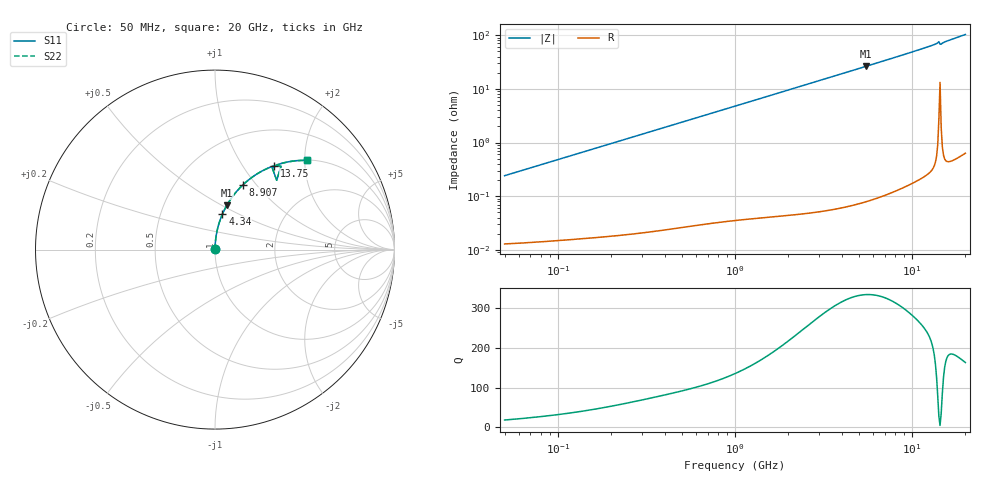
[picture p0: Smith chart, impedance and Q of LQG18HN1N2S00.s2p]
!Murata Part Number: LQG18HN1N2S00
!These Parameters are Measured in Series Mode Connection
!  o--[Z]--o
!Port1  Port2
!  o-------o
!Freq. Start=50[MHz] Stop=20[GHz], 401[Steps]
# Hz S RI R 50
!Freq.(Hz) S11(Real) S11(Imag) S21(Real) S21(Imag) S12(Real) S12(Imag) S22(Real) S22(Imag)
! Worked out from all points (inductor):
!   401 points, 50 MHz to 20 GHz, reference 50 ohm
!   read as one part in series: L = 767 pH near 51.52 MHz
!   highest Q = 332 at 5.516 GHz (marker M1), where L = 760 pH
!   S11 on the Smith chart (normalised r, x): 50 MHz: 1.00, +0.00; 4.34 GHz: 1.00, +0.41; 8.907 GHz: 1.00, +0.86; 13.75 GHz: 1.01, +1.39; 20 GHz: 1.01, +2.06
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5e7  0.000135 0.00241  0.9999 -0.00241  0.9999 -0.00241  0.000135 0.00241
1.364002e8  0.000204 0.00654  0.9998 -0.00654  0.9998 -0.00654  0.000204 0.00654
3.721004e8  0.000543 0.0178  0.9995 -0.0178  0.9995 -0.0178  0.000543 0.0178
1e9  0.00261 0.0474  0.9974 -0.0474  0.9974 -0.0474  0.00261 0.0474
1.714689e9  0.007 0.0809  0.993 -0.0809  0.993 -0.0809  0.007 0.0809
2.728004e9  0.017 0.1274  0.983 -0.1274  0.983 -0.1274  0.017 0.1274
4.34015e9  0.0416 0.198  0.9584 -0.198  0.9584 -0.198  0.0416 0.198
5.515528e9  0.0655 0.2459  0.9345 -0.2459  0.9345 -0.2459  0.0655 0.2459
7.442007e9  0.114 0.3163  0.886 -0.3163  0.886 -0.3163  0.114 0.3163
8.907419e9  0.157 0.3621  0.843 -0.3621  0.843 -0.3621  0.157 0.3621
1.019291e10  0.1979 0.3966  0.8021 -0.3966  0.8021 -0.3966  0.1979 0.3966
1.166392e10  0.2473 0.4295  0.7527 -0.4295  0.7527 -0.4295  0.2473 0.4295
1.314879e10  0.301 0.4562  0.699 -0.4562  0.699 -0.4562  0.301 0.4562
1.375312e10  0.3281 0.4655  0.6719 -0.4655  0.6719 -0.4655  0.3281 0.4655
1.396067e10  0.3419 0.468  0.6581 -0.468  0.6581 -0.468  0.3419 0.468
1.460232e10  0.3198 0.4526  0.6802 -0.4526  0.6802 -0.4526  0.3198 0.4526
1.482269e10  0.3362 0.4666  0.6638 -0.4666  0.6638 -0.4666  0.3362 0.4666
1.504638e10  0.3481 0.4724  0.6519 -0.4724  0.6519 -0.4724  0.3481 0.4724
1.573793e10  0.3762 0.4816  0.6238 -0.4816  0.6238 -0.4816  0.3762 0.4816
1.696185e10  0.4188 0.4906  0.5812 -0.4906  0.5812 -0.4906  0.4188 0.4906
1.940974e10  0.4965 0.497  0.5035 -0.497  0.5035 -0.497  0.4965 0.497
2e10  0.5141 0.4967  0.4859 -0.4967  0.4859 -0.4967  0.5141 0.4967
